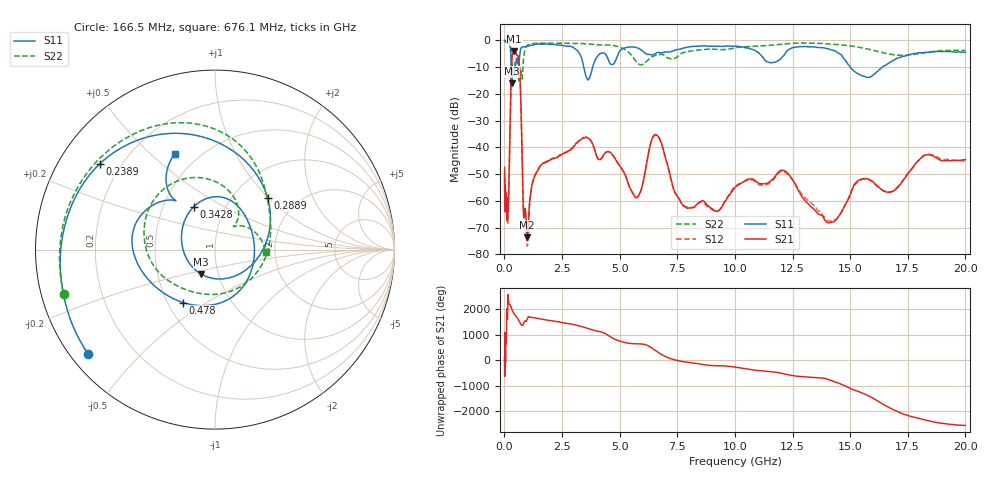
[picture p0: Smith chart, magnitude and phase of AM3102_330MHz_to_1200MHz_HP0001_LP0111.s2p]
! Date/Time: Tue, Sep 11, 2018 5:09 PM
! Network Analyzer: Agilent Technologies E8362B Rev: A.07.50.63
! Sweep from 0.010 to 20.000 GHz, 1601 Points, Sweep Type: LOG
! Power Supply: 4.949 V, 0.001 A
# Hz S DB R 50
!freq MagS11 AngS11 MagS21 AngS21 MagS12 AngS12 MagS22 AngS22
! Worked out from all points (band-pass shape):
!   1601 points, 10 MHz to 20 GHz, reference 50 ohm
!   highest |S21| = -4.02 dB at 420.4 MHz (marker M1); lowest = -73.6 dB at 993.4 MHz (marker M2)
!   |S21| within 3 dB of the highest: 324.7 MHz to 625.2 MHz (300.6 MHz wide, 63.3 % of centre)
!   lowest |S11| = -16.1 dB at 316.2 MHz (marker M3), VSWR 1.37, Z = 41.4 - j11.6 ohm
!   |S11| at or under -10 dB: 295.4 MHz to 464.4 MHz (169 MHz wide, 44.5 % of centre); 3.444 GHz to 3.828 GHz (385 MHz wide, 10.6 % of centre); 15.01 GHz to 16.4 GHz (1.392 GHz wide, 8.86 % of centre)
!   |S22| runs from -15.7 to -0.2 dB; largest |S21 - S12| = 0.011
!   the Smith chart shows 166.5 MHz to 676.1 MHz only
!   S11 on the Smith chart (normalised r, x): 166.5 MHz: 0.05, -0.36; 238.9 MHz: 0.12, +0.33; 288.9 MHz: 1.42, +0.99; 342.8 MHz: 0.71, +0.37; 478 MHz: 0.60, -0.40; 676.1 MHz: 0.37, +0.60
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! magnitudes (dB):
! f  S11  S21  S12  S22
! 10 MHz  0.0  -47.5  -52.5  -0.2
! 35.55 MHz  0.0  -59.3  -62.2  -0.4
! 126.4 MHz  -0.4  -65.1  -64.3  -0.9
! 166.5 MHz  -0.8  -64.3  -66.6  -1.1
! 238.9 MHz  -1.9  -36.8  -36.9  -1.8
! 288.9 MHz  -7.7  -15.2  -15.3  -3.7
! 316.2 MHz  -16.1  -8.1  -8.1  -7.0
! 342.8 MHz  -11.5  -5.7  -5.8  -10.0
! 420.4 MHz  -12.8  -4.0  -4.1  -10.6
! 447.2 MHz  -11.0  -4.2  -4.2  -9.1
! 478 MHz  -9.3  -4.4  -4.5  -7.9
! 676.1 MHz  -4.7  -13.7  -13.7  -11.0
! 829.3 MHz  -2.4  -64.6  -64.5  -7.0
! 993.4 MHz  -2.2  -73.6  -76.9  -1.9
! 1.59 GHz  -1.4  -46.6  -46.6  -1.0
! 3.582 GHz  -14.2  -36.3  -36.2  -1.3
! 5.652 GHz  -2.5  -58.3  -58.4  -7.1
! 6.58 GHz  -4.8  -35.3  -35.4  -5.5
! 7.882 GHz  -2.6  -62.5  -62.1  -4.3
! 12.09 GHz  -5.9  -48.6  -49.0  -1.3
! 14.01 GHz  -3.1  -68.2  -67.3  -1.3
! 20 GHz  -4.4  -44.5  -45.1  -3.7
